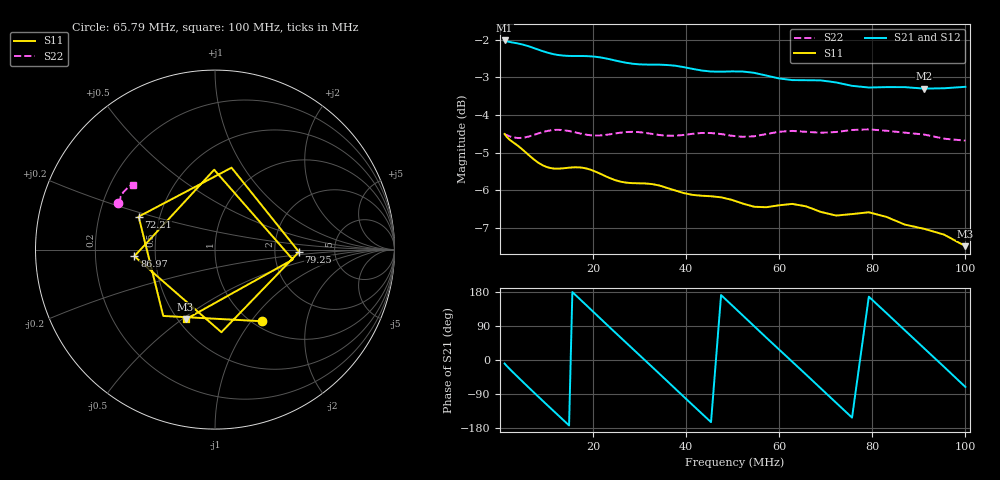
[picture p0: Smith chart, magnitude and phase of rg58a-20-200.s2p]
! ListType=Log
!!RG-58A/U 20' SWR=4 L=200
# MHZ S RI R 50
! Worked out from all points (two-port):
!   100 points, 1 MHz to 100 MHz, reference 50 ohm
!   highest |S21| = -2.02 dB at 1 MHz (marker M1); lowest = -3.3 dB at 91.12 MHz (marker M2)
!   |S21| within 3 dB of the highest: start of sweep to end of sweep
!   lowest |S11| = -7.5 dB at 100 MHz (marker M3), VSWR 2.46, Z = 27.3 - j25.8 ohm
!   |S11| at or under -10 dB: nowhere
!   |S22| runs from -4.7 to -4.4 dB; largest |S21 - S12| = 0.0032
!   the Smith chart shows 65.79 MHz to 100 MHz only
!   S11 on the Smith chart (normalised r, x): 65.79 MHz: 1.09, -1.13; 72.21 MHz: 0.38, +0.18; 79.25 MHz: 2.76, -0.09; 86.97 MHz: 0.38, -0.04; 100 MHz: 0.55, -0.52
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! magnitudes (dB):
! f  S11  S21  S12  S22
! 1 MHz  -4.5  -2.0  -2.0  -4.5
! 4.642 MHz  -4.9  -2.1  -2.1  -4.6
! 9.77 MHz  -5.4  -2.3  -2.3  -4.4
! 12.92 MHz  -5.4  -2.4  -2.4  -4.4
! 17.89 MHz  -5.4  -2.4  -2.4  -4.5
! 21.54 MHz  -5.6  -2.5  -2.5  -4.5
! 25.95 MHz  -5.8  -2.6  -2.6  -4.5
! 29.84 MHz  -5.8  -2.7  -2.6  -4.5
! 34.3 MHz  -5.9  -2.7  -2.7  -4.5
! 39.44 MHz  -6.1  -2.7  -2.7  -4.5
! 45.35 MHz  -6.2  -2.8  -2.8  -4.5
! 52.14 MHz  -6.4  -2.8  -2.9  -4.6
! 54.62 MHz  -6.4  -2.9  -2.9  -4.6
! 62.8 MHz  -6.4  -3.1  -3.1  -4.4
! 65.79 MHz  -6.4  -3.1  -3.1  -4.4
! 68.93 MHz  -6.6  -3.1  -3.1  -4.5
! 72.21 MHz  -6.7  -3.1  -3.1  -4.5
! 79.25 MHz  -6.6  -3.3  -3.3  -4.4
! 86.97 MHz  -6.9  -3.3  -3.3  -4.5
! 91.12 MHz  -7.0  -3.3  -3.3  -4.5
! 95.45 MHz  -7.2  -3.3  -3.3  -4.6
! 100 MHz  -7.5  -3.3  -3.2  -4.7
